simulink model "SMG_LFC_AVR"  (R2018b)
settings: Solver=VariableStepAuto  StartTime=0.0  StopTime=20  RelTol=1e-3
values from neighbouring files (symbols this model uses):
  D = 0.012    [System_Init.m]
  Ka = 10    [System_Init.m]
  Kbess = 1    [System_Init.m]
  Kc = 1    [System_Init.m]
  Kd = 1    [System_Init.m]
  Ke = 1    [System_Init.m]
  Kfc = 1    [System_Init.m]
  Kfess = 1    [System_Init.m]
  Kfilt1 = 1    [System_Init.m]
  Kg1 = 1    [System_Init.m]
  Kg2 = 1    [System_Init.m]
  Kh = 1    [System_Init.m]
  Kinv1 = 1    [System_Init.m]
  Kinv2 = 1    [System_Init.m]
  Ks = 1    [System_Init.m]
  M = 0.2    [System_Init.m]
  R = 3    [System_Init.m]
  Ta = 0.1    [System_Init.m]
  Tbess = 0.1    [System_Init.m]
  Tc = 0.5    [System_Init.m]
  Td = 0.4    [System_Init.m]
  Tdl = 1.0    (= 1)    [System_Init.m]
  Te = 0.4    [System_Init.m]
  TF = 0    [System_Init.m]
  Tfc = 0.26    [System_Init.m]
  Tfess = 0.1    [System_Init.m]
  Tfilt1 = 0.004    [System_Init.m]
  Tg1 = 0.08    [System_Init.m]
  Tg2 = 0.5    [System_Init.m]
  Th = 4    [System_Init.m]
  Tinv1 = 0.04    [System_Init.m]
  Tinv2 = 4    [System_Init.m]
  Ts = 0.05    [System_Init.m]
undefined symbols (not defined in the file or in its folder): b1, b2, K2, K4, K5, K6, Kd1, Kd2, Ki1, Ki2, Kp1, Kp2, N1, N2, Ps
libraries: simulink x4, cstblocks x2

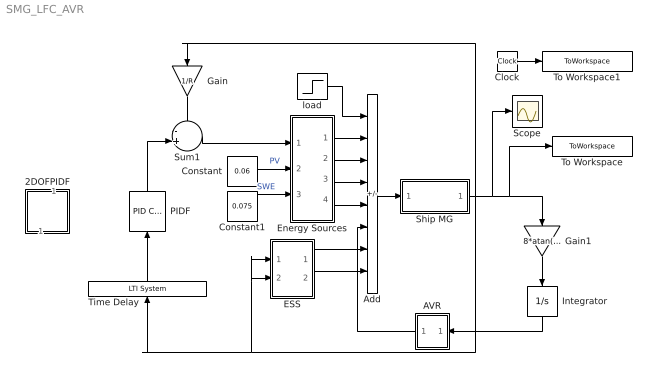
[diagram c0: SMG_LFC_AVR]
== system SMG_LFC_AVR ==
  2DOFPIDF : Subsystem  Commented=on
  AVR : Subsystem
  Add : Sum  Inputs=-++++---
  Clock : Clock
  Constant : Constant  Value=0.06  SampleTime=0
  Constant1 : Constant  Value=0.075  SampleTime=0
  ESS : Subsystem
  Energy Sources : Subsystem
  Gain : Gain  Gain=1/R
  Gain1 : Gain  Gain=8*atan(1.0)
  Integrator : Integrator
  PIDF : simulink/Continuous/PID Controller  Controller=PID  Form=Parallel  TimeDomain=Continuous-time  SampleTime=-1  IntegratorMethod=Forward Euler  ControllerParametersSource=internal  P=Kp1  I=Ki1  D=Kd1  UseFilter=on  N=N1  TunerSelectOption=Transfer Function Based (PID Tuner App)  InitialConditionSource=internal  InitialConditionForIntegrator=0  InitialConditionForFilter=0  DifferentiatorICPrevScaledInput=0  ExternalReset=none  TrackingMode=off  Kt=1  LimitOutput=off  UpperSaturationLimit=inf  LowerSaturationLimit=-inf  LinearizeAsGain=on  AntiWindupMode=none  Kb=1  POutMin=[]  POutMax=[]  IOutMin=[]  IOutMax=[]  DOutMin=[]  DOutMax=[]  NOutMin=[]  NOutMax=[]  SumOutMin=[]  SumOutMax=[]  SaturationOutMin=[]  SaturationOutMax=[]  PParamMin=[]  PParamMax=[]  IParamMin=[]  IParamMax=[]  DParamMin=[]  DParamMax=[]  NParamMin=[]  NParamMax=[]  KbParamMin=[]  KbParamMax=[]  KtParamMin=[]  KtParamMax=[]  KbOutMin=[]  KbOutMax=[]  KtOutMin=[]  KtOutMax=[]  IntegratorOutMin=[]  IntegratorOutMax=[]  FilterOutMin=[]  FilterOutMax=[]  SumI1OutMin=[]  SumI1OutMax=[]  SumI2OutMin=[]  SumI2OutMax=[]  SumI3OutMin=[]  SumI3OutMax=[]  SumI4OutMin=[]  SumI4OutMax=[]  SumDOutMin=[]  SumDOutMax=[]  DifferentiatorOutMin=[]  DifferentiatorOutMax=[]  FilterDiffOutCoefMin=[]  FilterDiffOutCoefMax=[]  ReciprocalOutMin=[]  ReciprocalOutMax=[]  SumDenOutMin=[]  SumDenOutMax=[]  SumNumOutMin=[]  SumNumOutMax=[]  DivideOutMin=[]  DivideOutMax=[]  IntegratorContinuousStateAttributes=''  IntegratorStateMustResolveToSignalObject=off  IntegratorRTWStateStorageClass=Auto  FilterContinuousStateAttributes=''  FilterStateMustResolveToSignalObject=off  FilterRTWStateStorageClass=Auto  ParallelPVariant=InternalParameters  IdealPVariant=Disabled  IVariant=InternalParameters  DVariant=InternalParameters  IntegratorVariant=Continuous  SatVariant=Disabled  AWVariant=Passthrough  PCopyVariant=Disabled  TRVariant=Disabled  FdbkBlocksVariant=Forward  IdealPFdbkVariant=Disabled  SatFdbkVariant=Disabled  DerivativeFilterVariant=ContFilter  NVariant=InternalParameters  NCopyVariant=Disabled  FilterICVariant=InternalICsFilter  IntegratorICVariant=InternalICs  ExternalResetVariant=Disabled  TRSumVariant=Passthrough  SumFdbkVariant=Disabled  SumVariant=Sum_PID
  Scope : Scope
  Ship MG : Subsystem
  Sum1 : Sum  Inputs=-+|
  Time Delay : cstblocks/LTI System  sys=tf(1,[TF 1],'InputDelay',Tdl)  IC=[]
  To Workspace : ToWorkspace  VariableName=Df  SampleTime=-1
  To Workspace1 : ToWorkspace  VariableName=Tsim  SampleTime=-1
  load : Step  Time=0  After=0.1  SampleTime=0
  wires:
  Add/1 -> Ship MG/1(In1)
  Gain1/1 -> Integrator/1
  Gain/1 -> Sum1/1
  Clock/1 -> To Workspace1/1
  Integrator/1 -> AVR/1(In1)
  Energy Sources/1(Out1) -> Add/2
  Energy Sources/3(Out3) -> Add/4
  Energy Sources/4(Out4) -> Add/5
  Energy Sources/2(Out2) -> Add/3
  Sum1/1 -> Energy Sources/1(In1)
  Constant/1 -> Energy Sources/2(In2)  "PV"
  Constant1/1 -> Energy Sources/3(In3)  "SWE"
  Time Delay/1 -> PIDF/1
  PIDF/1 -> Sum1/2
  Ship MG/1(Out1) -> Gain/1, Scope/1, To Workspace/1, Gain1/1, ESS/1(In1), ESS/2(In2), Time Delay/1
  ESS/1(Out1) -> Add/7
  ESS/2(Out2) -> Add/8
  AVR/1(Out1) -> Add/6
  load/1 -> Add/1

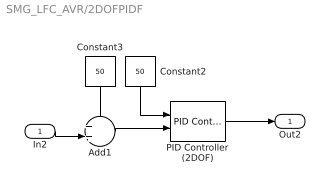
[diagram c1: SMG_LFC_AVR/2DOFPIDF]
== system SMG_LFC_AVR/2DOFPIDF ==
  In2 : Inport
  Add1 : Sum  Inputs=++|
  Constant2 : Constant  Value=50  SampleTime=0
  Constant3 : Constant  Value=50  SampleTime=0
  PID Controller (2DOF) : simulink/Continuous/PID Controller (2DOF)  Controller=PID  Form=Parallel  TimeDomain=Continuous-time  SampleTime=-1  IntegratorMethod=Forward Euler  ControllerParametersSource=internal  P=Kp1  I=Ki1  D=Kd1  UseFilter=on  N=N1  b=b1  c=c1  TunerSelectOption=Transfer Function Based (PID Tuner App)  InitialConditionSource=internal  InitialConditionForIntegrator=0  InitialConditionForFilter=0  DifferentiatorICPrevScaledInput=0  ExternalReset=none  TrackingMode=off  Kt=1  LimitOutput=off  UpperSaturationLimit=inf  LowerSaturationLimit=-inf  LinearizeAsGain=on  AntiWindupMode=none  Kb=1  POutMin=[]  POutMax=[]  IOutMin=[]  IOutMax=[]  DOutMin=[]  DOutMax=[]  NOutMin=[]  NOutMax=[]  bOutMin=[]  bOutMax=[]  cOutMin=[]  cOutMax=[]  SumOutMin=[]  SumOutMax=[]  SaturationOutMin=[]  SaturationOutMax=[]  PParamMin=[]  PParamMax=[]  IParamMin=[]  IParamMax=[]  DParamMin=[]  DParamMax=[]  NParamMin=[]  NParamMax=[]  bParamMin=[]  bParamMax=[]  cParamMin=[]  cParamMax=[]  KbParamMin=[]  KbParamMax=[]  KtParamMin=[]  KtParamMax=[]  KbOutMin=[]  KbOutMax=[]  KtOutMin=[]  KtOutMax=[]  IntegratorOutMin=[]  IntegratorOutMax=[]  FilterOutMin=[]  FilterOutMax=[]  SumI1OutMin=[]  SumI1OutMax=[]  SumI2OutMin=[]  SumI2OutMax=[]  SumI3OutMin=[]  SumI3OutMax=[]  SumI4OutMin=[]  SumI4OutMax=[]  SumDOutMin=[]  SumDOutMax=[]  Sum1OutMin=[]  Sum1OutMax=[]  Sum2OutMin=[]  Sum2OutMax=[]  Sum3OutMin=[]  Sum3OutMax=[]  DifferentiatorOutMin=[]  DifferentiatorOutMax=[]  FilterDiffOutCoefMin=[]  FilterDiffOutCoefMax=[]  ReciprocalOutMin=[]  ReciprocalOutMax=[]  SumDenOutMin=[]  SumDenOutMax=[]  SumNumOutMin=[]  SumNumOutMax=[]  DivideOutMin=[]  DivideOutMax=[]  IntegratorContinuousStateAttributes=''  IntegratorStateMustResolveToSignalObject=off  IntegratorRTWStateStorageClass=Auto  FilterContinuousStateAttributes=''  FilterStateMustResolveToSignalObject=off  FilterRTWStateStorageClass=Auto  ParallelPVariant=InternalParameters  IdealPVariant=Disabled  IVariant=InternalParameters  DVariant=InternalParameters  bVariant=InternalParameters  cVariant=InternalParameters  IntegratorVariant=Continuous  SatVariant=Disabled  AWVariant=Passthrough  PCopyVariant=Disabled  TRVariant=Disabled  FdbkBlocksVariant=Forward  IdealPFdbkVariant=Disabled  SatFdbkVariant=Disabled  DerivativeFilterVariant=ContFilter  NVariant=InternalParameters  NCopyVariant=Disabled  FilterICVariant=InternalICsFilter  IntegratorICVariant=InternalICs  ExternalResetVariant=Disabled  TRSumVariant=Passthrough  SumFdbkVariant=Disabled  SumVariant=Sum_PID
  Out2 : Outport
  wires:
  Add1/1 -> PID Controller (2DOF)/2
  Constant2/1 -> PID Controller (2DOF)/1
  PID Controller (2DOF)/1 -> Out2/1
  In2/1 -> Add1/2
  Constant3/1 -> Add1/1

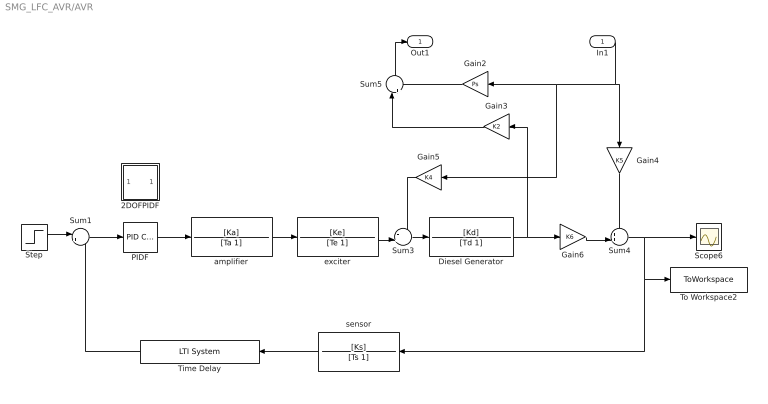
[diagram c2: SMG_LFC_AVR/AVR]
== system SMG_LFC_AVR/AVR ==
  In1 : Inport
  2DOFPIDF : Subsystem  Commented=on
  Diesel Generator : TransferFcn  Numerator=[Kd]  Denominator=[Td 1]
  Gain2 : Gain  Gain=Ps
  Gain3 : Gain  Gain=K2
  Gain4 : Gain  Gain=K5
  Gain5 : Gain  Gain=K4
  Gain6 : Gain  Gain=K6
  PIDF : simulink/Continuous/PID Controller  Controller=PID  Form=Parallel  TimeDomain=Continuous-time  SampleTime=-1  IntegratorMethod=Forward Euler  ControllerParametersSource=internal  P=Kp2  I=Ki2  D=Kd2  UseFilter=on  N=N2  TunerSelectOption=Transfer Function Based (PID Tuner App)  InitialConditionSource=internal  InitialConditionForIntegrator=0  InitialConditionForFilter=0  DifferentiatorICPrevScaledInput=0  ExternalReset=none  TrackingMode=off  Kt=1  LimitOutput=off  UpperSaturationLimit=inf  LowerSaturationLimit=-inf  LinearizeAsGain=on  AntiWindupMode=none  Kb=1  POutMin=[]  POutMax=[]  IOutMin=[]  IOutMax=[]  DOutMin=[]  DOutMax=[]  NOutMin=[]  NOutMax=[]  SumOutMin=[]  SumOutMax=[]  SaturationOutMin=[]  SaturationOutMax=[]  PParamMin=[]  PParamMax=[]  IParamMin=[]  IParamMax=[]  DParamMin=[]  DParamMax=[]  NParamMin=[]  NParamMax=[]  KbParamMin=[]  KbParamMax=[]  KtParamMin=[]  KtParamMax=[]  KbOutMin=[]  KbOutMax=[]  KtOutMin=[]  KtOutMax=[]  IntegratorOutMin=[]  IntegratorOutMax=[]  FilterOutMin=[]  FilterOutMax=[]  SumI1OutMin=[]  SumI1OutMax=[]  SumI2OutMin=[]  SumI2OutMax=[]  SumI3OutMin=[]  SumI3OutMax=[]  SumI4OutMin=[]  SumI4OutMax=[]  SumDOutMin=[]  SumDOutMax=[]  DifferentiatorOutMin=[]  DifferentiatorOutMax=[]  FilterDiffOutCoefMin=[]  FilterDiffOutCoefMax=[]  ReciprocalOutMin=[]  ReciprocalOutMax=[]  SumDenOutMin=[]  SumDenOutMax=[]  SumNumOutMin=[]  SumNumOutMax=[]  DivideOutMin=[]  DivideOutMax=[]  IntegratorContinuousStateAttributes=''  IntegratorStateMustResolveToSignalObject=off  IntegratorRTWStateStorageClass=Auto  FilterContinuousStateAttributes=''  FilterStateMustResolveToSignalObject=off  FilterRTWStateStorageClass=Auto  ParallelPVariant=InternalParameters  IdealPVariant=Disabled  IVariant=InternalParameters  DVariant=InternalParameters  IntegratorVariant=Continuous  SatVariant=Disabled  AWVariant=Passthrough  PCopyVariant=Disabled  TRVariant=Disabled  FdbkBlocksVariant=Forward  IdealPFdbkVariant=Disabled  SatFdbkVariant=Disabled  DerivativeFilterVariant=ContFilter  NVariant=InternalParameters  NCopyVariant=Disabled  FilterICVariant=InternalICsFilter  IntegratorICVariant=InternalICs  ExternalResetVariant=Disabled  TRSumVariant=Passthrough  SumFdbkVariant=Disabled  SumVariant=Sum_PID
  Scope6 : Scope
  Step : Step  Time=0  Before=1  SampleTime=0
  Sum1 : Sum  Inputs=|+-
  Sum3 : Sum  Inputs=-+|
  Sum4 : Sum  Inputs=++|
  Sum5 : Sum  Inputs=|++
  Time Delay : cstblocks/LTI System  sys=tf(1,[TF 1],'InputDelay',Tdl)  IC=[]
  To Workspace2 : ToWorkspace  VariableName=Vbus  SampleTime=-1
  amplifier : TransferFcn  Numerator=[Ka]  Denominator=[Ta 1]
  exciter : TransferFcn  Numerator=[Ke]  Denominator=[Te 1]
  sensor : TransferFcn  Numerator=[Ks]  Denominator=[Ts 1]
  Out1 : Outport
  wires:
  Gain6/1 -> Sum4/2
  amplifier/1 -> exciter/1
  In1/1 -> Gain5/1, Gain2/1, Gain4/1
  Sum5/1 -> Out1/1
  Gain4/1 -> Sum4/1
  Gain5/1 -> Sum3/1
  Sum4/1 -> Scope6/1, To Workspace2/1, sensor/1
  Sum3/1 -> Diesel Generator/1
  Gain2/1 -> Sum5/2
  exciter/1 -> Sum3/2
  Gain3/1 -> Sum5/1
  Diesel Generator/1 -> Gain3/1, Gain6/1
  PIDF/1 -> amplifier/1
  Step/1 -> Sum1/1
  Sum1/1 -> PIDF/1
  sensor/1 -> Time Delay/1
  Time Delay/1 -> Sum1/2

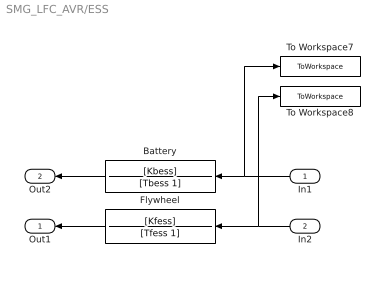
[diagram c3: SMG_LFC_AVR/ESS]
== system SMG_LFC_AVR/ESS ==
  In1 : Inport
  In2 : Inport  Port=2
  Battery : TransferFcn  Numerator=[Kbess]  Denominator=[Tbess 1]
  Flywheel : TransferFcn  Numerator=[Kfess]  Denominator=[Tfess 1]
  To Workspace7 : ToWorkspace  VariableName=Battery  SaveFormat=Structure  SampleTime=-1
  To Workspace8 : ToWorkspace  VariableName=Flywheel  SaveFormat=Structure  SampleTime=-1
  Out1 : Outport
  Out2 : Outport  Port=2
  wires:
  Battery/1 -> Out2/1
  In2/1 -> To Workspace8/1, Flywheel/1
  In1/1 -> To Workspace7/1, Battery/1
  Flywheel/1 -> Out1/1

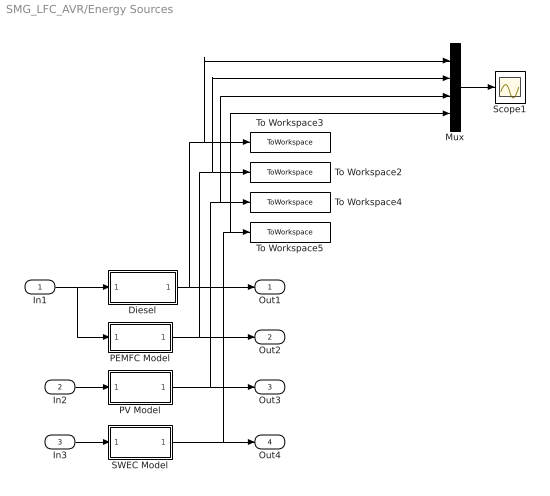
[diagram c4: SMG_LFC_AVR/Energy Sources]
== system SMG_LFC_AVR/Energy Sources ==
  In1 : Inport
  In2 : Inport  Port=2
  In3 : Inport  Port=3
  Diesel : Subsystem
  Mux : Mux
  PEMFC Model : Subsystem
  PV Model : Subsystem
  SWEC Model : Subsystem
  Scope1 : Scope
  To Workspace2 : ToWorkspace  VariableName=PEMFC  SaveFormat=Structure  SampleTime=-1
  To Workspace3 : ToWorkspace  VariableName=Diesel  SaveFormat=Structure  SampleTime=-1
  To Workspace4 : ToWorkspace  VariableName=PV  SaveFormat=Structure  SampleTime=-1
  To Workspace5 : ToWorkspace  VariableName=SWEC  SaveFormat=Structure  SampleTime=-1
  Out1 : Outport
  Out2 : Outport  Port=2
  Out3 : Outport  Port=3
  Out4 : Outport  Port=4
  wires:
  In2/1 -> PV Model/1(In1)
  In1/1 -> PEMFC Model/1(In1), Diesel/1(In1)
  PV Model/1(Out1) -> To Workspace4/1, Mux/3, Out3/1
  PEMFC Model/1(Out1) -> To Workspace2/1, Mux/2, Out2/1
  SWEC Model/1(Out1) -> Mux/4, To Workspace5/1, Out4/1
  Diesel/1(Out1) -> Mux/1, To Workspace3/1, Out1/1
  In3/1 -> SWEC Model/1(In1)
  Mux/1 -> Scope1/1

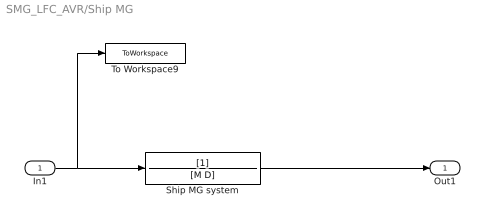
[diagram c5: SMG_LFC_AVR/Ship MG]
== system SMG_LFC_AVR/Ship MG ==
  In1 : Inport
  Ship MG system : TransferFcn  Denominator=[M D]
  To Workspace9 : ToWorkspace  VariableName=isozygio  SaveFormat=Structure  SampleTime=-1
  Out1 : Outport
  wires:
  Ship MG system/1 -> Out1/1
  In1/1 -> To Workspace9/1, Ship MG system/1

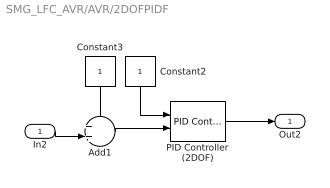
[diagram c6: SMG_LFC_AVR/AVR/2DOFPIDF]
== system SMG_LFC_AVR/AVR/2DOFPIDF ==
  In2 : Inport
  Add1 : Sum  Inputs=++|
  Constant2 : Constant  SampleTime=0
  Constant3 : Constant  SampleTime=0
  PID Controller (2DOF) : simulink/Continuous/PID Controller (2DOF)  Controller=PID  Form=Parallel  TimeDomain=Continuous-time  SampleTime=-1  IntegratorMethod=Forward Euler  ControllerParametersSource=internal  P=Kp2  I=Ki2  D=Kd2  UseFilter=on  N=N2  b=b2  c=c2  TunerSelectOption=Transfer Function Based (PID Tuner App)  InitialConditionSource=internal  InitialConditionForIntegrator=0  InitialConditionForFilter=0  DifferentiatorICPrevScaledInput=0  ExternalReset=none  TrackingMode=off  Kt=1  LimitOutput=off  UpperSaturationLimit=inf  LowerSaturationLimit=-inf  LinearizeAsGain=on  AntiWindupMode=none  Kb=1  POutMin=[]  POutMax=[]  IOutMin=[]  IOutMax=[]  DOutMin=[]  DOutMax=[]  NOutMin=[]  NOutMax=[]  bOutMin=[]  bOutMax=[]  cOutMin=[]  cOutMax=[]  SumOutMin=[]  SumOutMax=[]  SaturationOutMin=[]  SaturationOutMax=[]  PParamMin=[]  PParamMax=[]  IParamMin=[]  IParamMax=[]  DParamMin=[]  DParamMax=[]  NParamMin=[]  NParamMax=[]  bParamMin=[]  bParamMax=[]  cParamMin=[]  cParamMax=[]  KbParamMin=[]  KbParamMax=[]  KtParamMin=[]  KtParamMax=[]  KbOutMin=[]  KbOutMax=[]  KtOutMin=[]  KtOutMax=[]  IntegratorOutMin=[]  IntegratorOutMax=[]  FilterOutMin=[]  FilterOutMax=[]  SumI1OutMin=[]  SumI1OutMax=[]  SumI2OutMin=[]  SumI2OutMax=[]  SumI3OutMin=[]  SumI3OutMax=[]  SumI4OutMin=[]  SumI4OutMax=[]  SumDOutMin=[]  SumDOutMax=[]  Sum1OutMin=[]  Sum1OutMax=[]  Sum2OutMin=[]  Sum2OutMax=[]  Sum3OutMin=[]  Sum3OutMax=[]  DifferentiatorOutMin=[]  DifferentiatorOutMax=[]  FilterDiffOutCoefMin=[]  FilterDiffOutCoefMax=[]  ReciprocalOutMin=[]  ReciprocalOutMax=[]  SumDenOutMin=[]  SumDenOutMax=[]  SumNumOutMin=[]  SumNumOutMax=[]  DivideOutMin=[]  DivideOutMax=[]  IntegratorContinuousStateAttributes=''  IntegratorStateMustResolveToSignalObject=off  IntegratorRTWStateStorageClass=Auto  FilterContinuousStateAttributes=''  FilterStateMustResolveToSignalObject=off  FilterRTWStateStorageClass=Auto  ParallelPVariant=InternalParameters  IdealPVariant=Disabled  IVariant=InternalParameters  DVariant=InternalParameters  bVariant=InternalParameters  cVariant=InternalParameters  IntegratorVariant=Continuous  SatVariant=Disabled  AWVariant=Passthrough  PCopyVariant=Disabled  TRVariant=Disabled  FdbkBlocksVariant=Forward  IdealPFdbkVariant=Disabled  SatFdbkVariant=Disabled  DerivativeFilterVariant=ContFilter  NVariant=InternalParameters  NCopyVariant=Disabled  FilterICVariant=InternalICsFilter  IntegratorICVariant=InternalICs  ExternalResetVariant=Disabled  TRSumVariant=Passthrough  SumFdbkVariant=Disabled  SumVariant=Sum_PID
  Out2 : Outport
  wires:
  Add1/1 -> PID Controller (2DOF)/2
  Constant2/1 -> PID Controller (2DOF)/1
  PID Controller (2DOF)/1 -> Out2/1
  In2/1 -> Add1/2
  Constant3/1 -> Add1/1

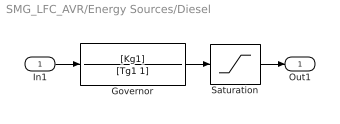
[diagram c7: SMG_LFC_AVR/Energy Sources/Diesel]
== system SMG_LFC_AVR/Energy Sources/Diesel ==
  In1 : Inport
  Governor : TransferFcn  Numerator=[Kg1]  Denominator=[Tg1 1]
  Saturation : Saturate  UpperLimit=0.05  LowerLimit=-0.05
  Out1 : Outport
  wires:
  In1/1 -> Governor/1
  Governor/1 -> Saturation/1
  Saturation/1 -> Out1/1

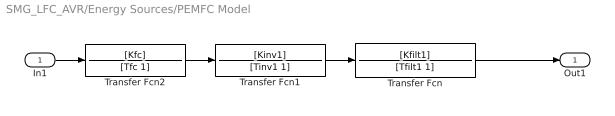
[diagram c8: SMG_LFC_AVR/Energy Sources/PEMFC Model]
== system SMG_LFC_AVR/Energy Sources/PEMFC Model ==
  In1 : Inport
  Transfer Fcn : TransferFcn  Numerator=[Kfilt1]  Denominator=[Tfilt1 1]
  Transfer Fcn1 : TransferFcn  Numerator=[Kinv1]  Denominator=[Tinv1 1]
  Transfer Fcn2 : TransferFcn  Numerator=[Kfc]  Denominator=[Tfc 1]
  Out1 : Outport
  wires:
  Transfer Fcn1/1 -> Transfer Fcn/1
  In1/1 -> Transfer Fcn2/1
  Transfer Fcn2/1 -> Transfer Fcn1/1
  Transfer Fcn/1 -> Out1/1

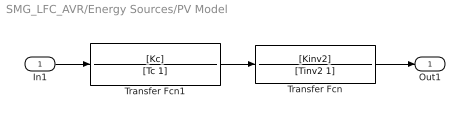
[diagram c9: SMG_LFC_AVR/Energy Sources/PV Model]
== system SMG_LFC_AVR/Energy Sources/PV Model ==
  In1 : Inport
  Transfer Fcn : TransferFcn  Numerator=[Kinv2]  Denominator=[Tinv2 1]
  Transfer Fcn1 : TransferFcn  Numerator=[Kc]  Denominator=[Tc 1]
  Out1 : Outport
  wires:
  In1/1 -> Transfer Fcn1/1
  Transfer Fcn1/1 -> Transfer Fcn/1
  Transfer Fcn/1 -> Out1/1

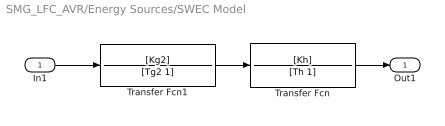
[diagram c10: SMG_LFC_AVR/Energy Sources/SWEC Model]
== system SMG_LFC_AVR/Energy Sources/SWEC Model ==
  In1 : Inport
  Transfer Fcn : TransferFcn  Numerator=[Kh]  Denominator=[Th 1]
  Transfer Fcn1 : TransferFcn  Numerator=[Kg2]  Denominator=[Tg2 1]
  Out1 : Outport
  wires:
  Transfer Fcn1/1 -> Transfer Fcn/1
  In1/1 -> Transfer Fcn1/1
  Transfer Fcn/1 -> Out1/1
